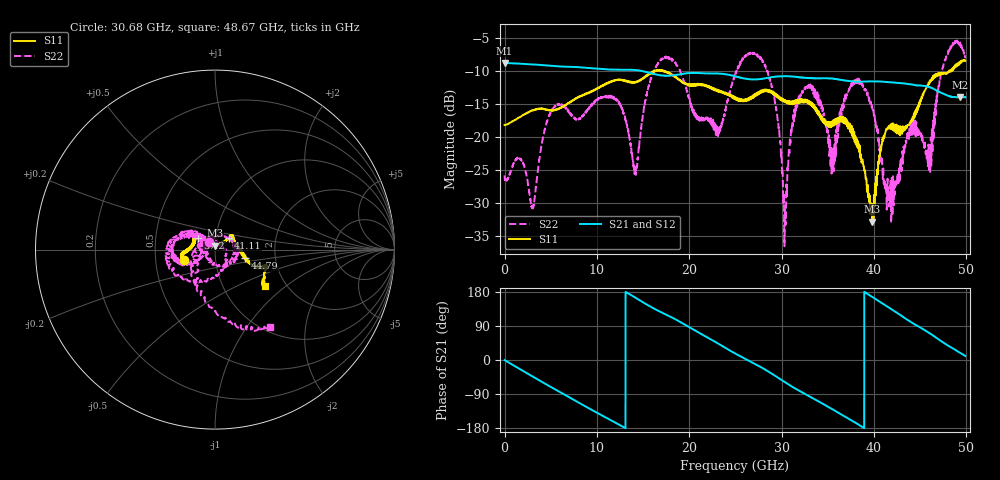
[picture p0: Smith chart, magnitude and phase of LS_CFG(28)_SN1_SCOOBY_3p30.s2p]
!Keysight Technologies,N5245B,MY58422026,A.13.80.08
!Date: Thursday, March 19, 2020 23:35:31
!Correction: S11(Full 2 Port(1,2))
!S21(Full 2 Port(1,2))
!S12(Full 2 Port(1,2))
!S22(Full 2 Port(1,2))
!S2P File: Measurements: S11, S21, S12, S22:
# Hz S DB R 50.0
!freq dBS11 angS11 dBS21 angS21 dBS12 angS12 dBS22 angS22
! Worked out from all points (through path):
!   4991 points, 10 MHz to 49.91 GHz, reference 50 ohm
!   highest |S21| = -8.74 dB at 10 MHz (marker M1); lowest = -14.0 dB at 49.34 GHz (marker M2)
!   group delay of S21, straight-line fit = 39 ps
!   lowest |S11| = -32.9 dB at 39.84 GHz (marker M3), VSWR 1.05, Z = 49.9 + j2.28 ohm
!   |S11| at or under -10 dB: start of sweep to 16.08 GHz; 16.09 GHz to 16.17 GHz (85.95 MHz wide, 0.533 % of centre); 17.42 GHz to 48.16 GHz (30.74 GHz wide, 93.8 % of centre)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
!   |S22| runs from -36.6 to -5.3 dB; largest |S21 - S12| = 0.0036
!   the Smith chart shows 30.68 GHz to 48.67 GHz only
!   S11 on the Smith chart (normalised r, x): 30.68 GHz: 0.70, -0.09; 37.2 GHz: 0.82, +0.11; 41.11 GHz: 1.15, +0.15; 44.79 GHz: 1.39, -0.13; 48.67 GHz: 1.56, -0.72
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1e7  -18.19 -1.7  -8.74 -0.3  -8.73 -0.3  -25.83 1.0
3.04e9  -15.96 -35.8  -8.98 -43.5  -8.97 -43.4  -31.07 -71.0
5.05e9  -15.97 -54.5  -9.19 -71.7  -9.19 -71.7  -16.08 -105.7
8.33e9  -13.79 -77.4  -9.43 -116.5  -9.43 -116.5  -17.00 -96.9
1.208e10  -11.35 -101.2  -9.78 -166.3  -9.78 -166.3  -14.18 -88.9
1.418e10  -11.65 -116.1  -9.83 164.4  -9.82 164.4  -25.24 -135.8
1.665e10  -9.89 -126.5  -10.57 129.8  -10.56 129.9  -8.76 -165.1
2.312e10  -13.11 -149.4  -10.35 43.5  -10.35 43.7  -19.86 -156.1
2.496e10  -14.11 -149.2  -10.75 17.4  -10.74 17.6  -10.66 -170.9
2.81e10  -12.89 -157.0  -11.12 -23.6  -11.12 -23.4  -8.82 -90.7
3.068e10  -14.68 -160.9  -10.76 -63.4  -10.76 -63.2  -25.03 129.0
3.328e10  -14.95 -175.9  -11.05 -99.7  -11.05 -99.4  -12.45 -168.1
3.553e10  -18.16 155.1  -11.12 -130.4  -11.06 -130.0  -25.53 177.1
3.72e10  -18.64 144.9  -11.48 -154.2  -11.40 -154.3  -13.15 158.3
3.984e10  -32.85 90.1  -11.55 166.2  -11.53 166.1  -15.75 -96.4
4.111e10  -20.11 40.3  -11.61 146.2  -11.62 146.1  -27.09 18.2
4.16e10  -18.34 40.0  -11.67 138.7  -11.70 138.5  -27.80 99.7
4.479e10  -15.30 -15.4  -12.15 89.0  -12.18 89.0  -19.29 15.9
4.601e10  -11.83 -23.3  -12.42 70.9  -12.44 70.9  -22.37 122.8
4.867e10  -9.30 -36.2  -13.96 28.8  -13.97 28.9  -5.53 -54.5
4.934e10  -8.71 -41.1  -13.99 18.8  -14.00 18.9  -5.64 -31.0
4.991e10  -8.40 -37.0  -13.94 10.5  -13.96 10.4  -7.85 -15.3
